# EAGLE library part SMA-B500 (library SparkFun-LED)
American Opto Plus LED Corp. - SMA-B520LB 5 segment SMD LED Bar Graph Display, Bright Blue SparkFun Products: MyoWare LED Shield
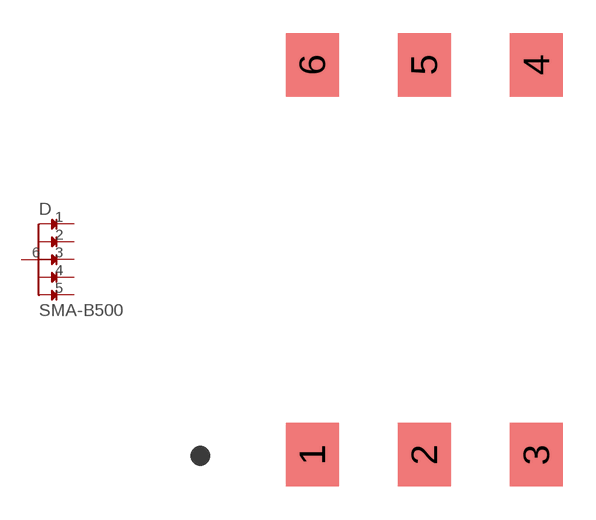
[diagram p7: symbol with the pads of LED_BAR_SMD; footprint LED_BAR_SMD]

Designator prefix D

## SMA-B500 (PROD_ID: DIO-13127)  [LED_BAR_SMD]
1  1
2  2
3  3
4  4
5  5
6  6

## Footprint LED_BAR_SMD (pad centres in mm)
SMA-B520LB LED Bargraph - 5 segment Specifications: Pin count:6 Datasheet referenced for footprint Example device(s): [EXAMPLE DEVICE 1] [EXAMPLE DEVICE 2]
smd 2.4 x 2.88: 1 -5.08,-8.84; 2 0,-8.84; 3 5.08,-8.84; 4 5.08,8.84; 5 0,8.84; 6 -5.08,8.84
